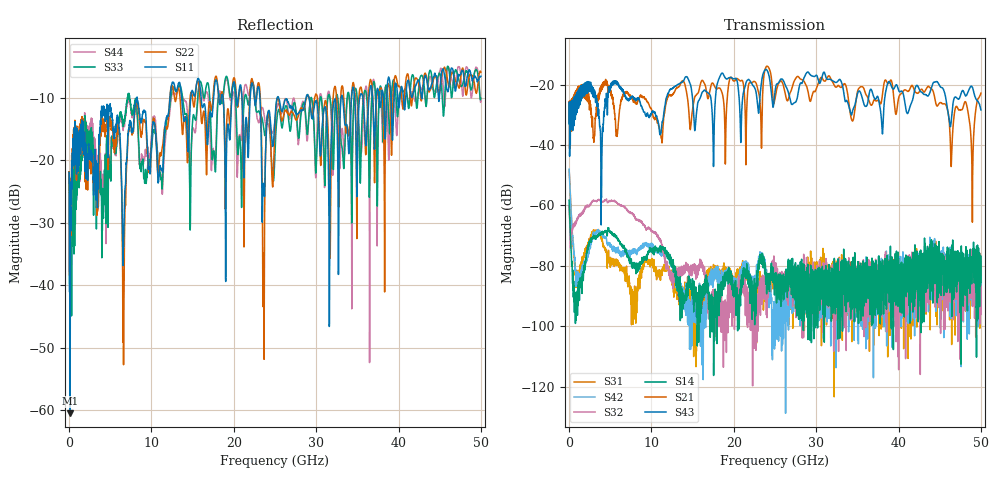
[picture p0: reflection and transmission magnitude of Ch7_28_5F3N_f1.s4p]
!Agilent Technologies,N5247A,US51170199,A.09.90.13
!Agilent N5247A: A.09.90.13
!Date: Wednesday, December 09, 2015 09:41:37
!Correction: S11(Full 4 Port(1,2,3,4))
!S12(Full 4 Port(1,2,3,4))
!S13(Full 4 Port(1,2,3,4))
!S14(Full 4 Port(1,2,3,4))
!S21(Full 4 Port(1,2,3,4))
!S22(Full 4 Port(1,2,3,4))
!S23(Full 4 Port(1,2,3,4))
!S24(Full 4 Port(1,2,3,4))
!S31(Full 4 Port(1,2,3,4))
!S32(Full 4 Port(1,2,3,4))
!S33(Full 4 Port(1,2,3,4))
!S34(Full 4 Port(1,2,3,4))
!S41(Full 4 Port(1,2,3,4))
!S42(Full 4 Port(1,2,3,4))
!S43(Full 4 Port(1,2,3,4))
!S44(Full 4 Port(1,2,3,4))
!S4P File: Measurements: <S11,S12,S13,S14>,
!<S21,S22,S23,S24>,
!<S31,S32,S33,S34>,
!<S41,S42,S43,S44>:
# Hz S  dB  R 50
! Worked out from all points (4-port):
!   3201 points, 10 MHz to 50 GHz, reference 50 ohm
!   strongest paths, dB at 10 MHz, 12.51 GHz, 25 GHz, 37.5 GHz, 50 GHz:
!     S43: -33.0, -21.3, -22.4, -24.1, -28.4
!     S21: -32.5, -23.5, -24.8, -25.2, -22.9
!     S14: -58.3, -78.3, -83.1, -95.9, -85.5
!     S32: -60.2, -84.0, -80.0, -82.6, -86.7
!     S42: -48.0, -79.9, -94.7, -83.8, -89.9
!     S31: -48.3, -84.4, -88.0, -84.4, -82.4
!   lowest |S11| = -60.5 dB at 135 MHz (marker M1), VSWR 1.00, Z = 50 + j0.0826 ohm
!   |S11| at or under -10 dB: start of sweep to 8.236 GHz; 8.271 GHz to 12.25 GHz (3.982 GHz wide, 38.8 % of centre); 29.14 GHz to 33.03 GHz (3.891 GHz wide, 12.5 % of centre)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
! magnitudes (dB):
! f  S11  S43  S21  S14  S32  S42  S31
! 10 MHz  -21.9  -33.0  -32.5  -58.3  -60.2  -48.0  -48.3
! 135 MHz  -60.5  -31.8  -32.8  -67.5  -72.5  -55.3  -55.2
! 978.6 MHz  -21.2  -25.7  -27.2  -94.2  -65.0  -86.7  -85.2
! 6.649 GHz  -31.8  -22.7  -23.4  -73.2  -60.1  -75.6  -81.3
! 8.196 GHz  -10.1  -25.0  -26.5  -80.9  -64.7  -75.1  -90.7
! 23.65 GHz  -24.2  -15.9  -17.4  -77.5  -85.7  -78.2  -90.2
! 50 GHz  -6.5  -28.4  -22.9  -85.5  -86.7  -89.9  -82.4
